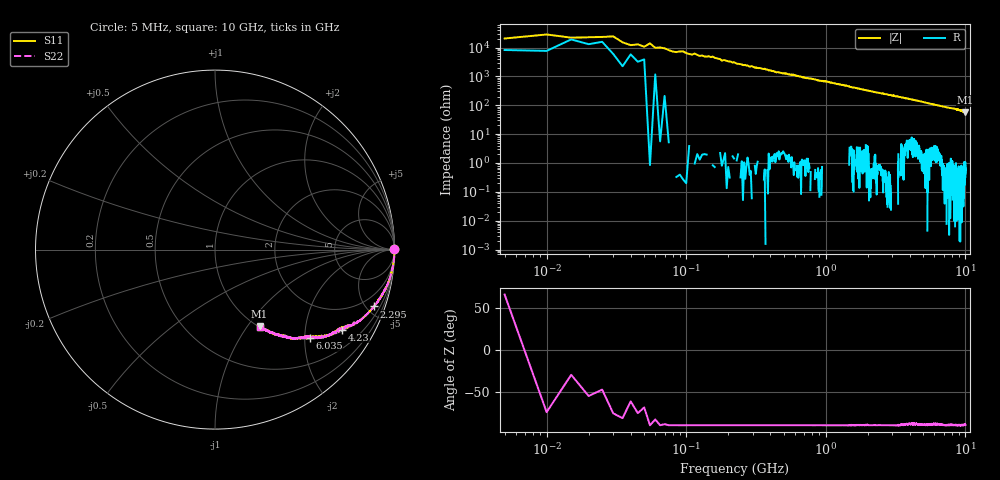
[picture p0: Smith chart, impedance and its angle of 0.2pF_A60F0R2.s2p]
! Amotech Co.,Ltd.
! http://www.amotech.co.kr/
! Part Number: A60F0R2
! These Parameters are Measured in Series Mode Connection
! Operation Temp=25[degC], DC Bias Voltage=0[V]
! Freq. Start=5[MHz] Stop=10[GHz], 2000[Steps]
! Date: Monday, July 20, 2020, 03:11:15
# GHZ S RI R 50.000000
!Freq.(Hz) S11(Real) S11(Imag) S21(Real) S21(Imag) S12(Real) S12(Imag) S22(Real) S22(Imag)
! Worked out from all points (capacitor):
!   2000 points, 5 MHz to 10 GHz, reference 50 ohm
!   read as one part in series: C = 249 fF near 55 MHz
!   lowest |Z| = 57.1 ohm at 9.98 GHz (marker M1)
!   S11 on the Smith chart (normalised r, x): 5 MHz: open; 2.295 GHz: 1.01, -5.60; 4.23 GHz: 1.06, -3.13; 6.035 GHz: 1.03, -2.11; 10 GHz: 1.01, -1.15
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0.005  0.998 0.00445  0.00196 -0.00445  0.00196 -0.00445  0.998 0.00445
0.02  0.9975 -0.00359  0.00254 0.00359  0.00254 0.00359  0.9975 -0.00359
0.045  0.998 -0.00751  0.002 0.00751  0.002 0.00751  0.998 -0.00751
0.085  0.9998 -0.0144  0.000208 0.0144  0.000208 0.0144  0.9998 -0.0144
0.11  0.9997 -0.0176  0.000306 0.0176  0.000306 0.0176  0.9997 -0.0176
0.15  0.9995 -0.0216  0.000463 0.0216  0.000463 0.0216  0.9995 -0.0216
0.21  0.999 -0.0312  0.000968 0.0312  0.000968 0.0312  0.999 -0.0312
0.28  0.998 -0.0447  0.00202 0.0447  0.00202 0.0447  0.998 -0.0447
0.455  0.9948 -0.0711  0.00517 0.0711  0.00517 0.0711  0.9948 -0.0711
0.69  0.9887 -0.1053  0.0113 0.1053  0.0113 0.1053  0.9887 -0.1053
0.9  0.9806 -0.1378  0.0194 0.1378  0.0194 0.1378  0.9806 -0.1378
1.24  0.9665 -0.1809  0.0335 0.1809  0.0335 0.1809  0.9665 -0.1809
1.675  0.9369 -0.2415  0.0631 0.2415  0.0631 0.2415  0.9369 -0.2415
2.295  0.8864 -0.3166  0.1136 0.3166  0.1136 0.3166  0.8864 -0.3166
3.34  0.7895 -0.4095  0.2105 0.4095  0.2105 0.4095  0.7895 -0.4095
4.23  0.7065 -0.4453  0.2935 0.4453  0.2935 0.4453  0.7065 -0.4453
5.005  0.6239 -0.4818  0.3761 0.4818  0.3761 0.4818  0.6239 -0.4818
6.035  0.5272 -0.4926  0.4728 0.4926  0.4728 0.4926  0.5272 -0.4926
6.67  0.47 -0.4927  0.53 0.4927  0.53 0.4927  0.47 -0.4927
8.335  0.3672 -0.4812  0.6328 0.4812  0.6328 0.4812  0.3672 -0.4812
9.98  0.248 -0.427  0.752 0.427  0.752 0.427  0.248 -0.427
10  0.2483 -0.4292  0.7517 0.4292  0.7517 0.4292  0.2483 -0.4292
